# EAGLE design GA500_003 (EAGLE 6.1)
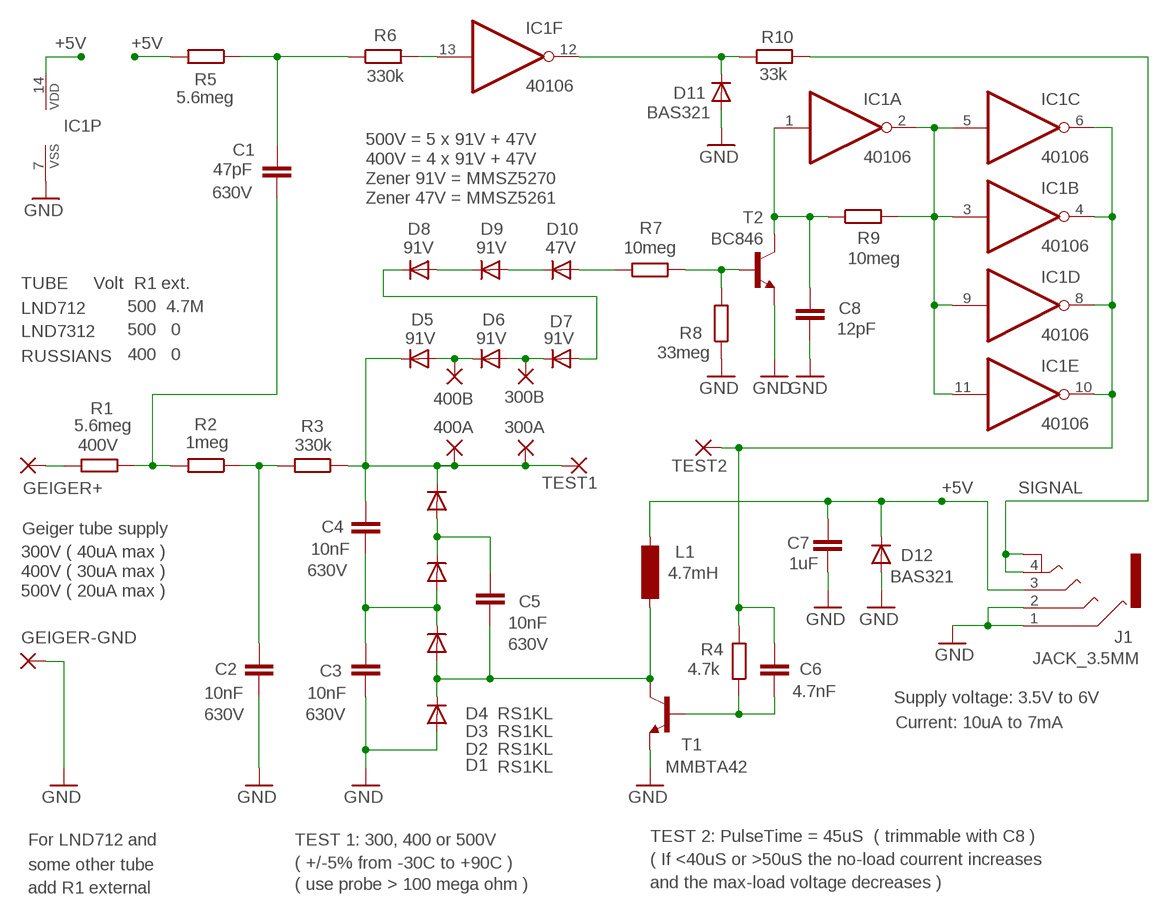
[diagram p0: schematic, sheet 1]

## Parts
300A  TEST  WIREPADSMD1,00-1,00  [SMD1,00-1,00]
300B  TEST  WIREPADSMD1,00-1,00  [SMD1,00-1,00]
400A  TEST  WIREPADSMD1,00-1,00  [SMD1,00-1,00]
400B  TEST  WIREPADSMD1,00-1,00  [SMD1,00-1,00]
C1  47pF  C-EUC1206  [C1206]
C2  10nF  C-EUC1206  [C1206]
C3  10nF  C-EUC1206  [C1206]
C4  10nF  C-EUC1206  [C1206]
C5  10nF  C-EUC1206  [C1206]
C6  4.7nF  C-EUC0603  [C0603]
C7  1uF  C-EUC0603  [C0603]
C8  12pF  C-EUC0603  [C0603]
D1  RS1KL  DIODE-SOD123-LARGE  [SOD123-LARGE]
D2  RS1KL  DIODE-SOD123-LARGE  [SOD123-LARGE]
D3  RS1KL  DIODE-SOD123-LARGE  [SOD123-LARGE]
D4  RS1KL  DIODE-SOD123-LARGE  [SOD123-LARGE]
D5  MMSZ5270  DIODE-SOD123  [SOD123]
D6  MMSZ5270  DIODE-SOD123  [SOD123]
D7  MMSZ5270  DIODE-SOD123  [SOD123]
D8  MMSZ5270  DIODE-SOD123  [SOD123]
D9  MMSZ5270  DIODE-SOD123  [SOD123]
D10  MMSZ5261  DIODE-SOD123-LARGE  [SOD123-LARGE]
D11  BAS321  DIODE-SOD323  [SOD323]
D12  BAS321  DIODE-SOD323  [SOD323]
GEIGER+  Geiger tube supply  WIREPADSMD2,54-3,81  [SMD2,54-3,81]
GEIGER-GND  1.6mm  WIREPADSMD2,54-3,81  [SMD2,54-3,81]
IC1  40106  40106SOIC  [SOIC14_S]
J1  JACK_3.5MM  JACK_3.5MM_SMD_4JACK4  [JACK_4]
L1  4.7mH  INDUCTOR_4.7MH472KU  [MSD75]
R1  5.6meg  R-EU_R1206  [R1206]
R2  1meg  R-EU_R1206  [R1206]
R3  330k  R-EU_R1206  [R1206]
R4  4.7k  R-EU_R0603  [R0603]
R5  5.6meg  R-EU_R1206  [R1206]
R6  330k  R-EU_R1206  [R1206]
R7  10meg  R-EU_R1206_L  [R1206_L]
R8  33meg  R-EU_R0603  [R0603]
R9  10meg  R-EU_R0603  [R0603]
R10  33k  R-EU_R0603  [R0603]
T1  MMBTA42  -NPN-BC846  [SOT23_L]
T2  BC846  BC846L  [SOT23_L]
TEST1  TEST  WIREPADSMD1,27-2,54  [SMD1,27-2,54]
TEST2  TEST  WIREPADSMD1,27-2,54  [SMD1,27-2,54]

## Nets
+5V: C7.1 D12.C IC1.14(P:VDD) J1.3 L1.1 R5.2
DATA: C1.1 R5.1 R6.1
GND: C2.1 C3.1 C7.2 C8.2 D1.A D11.A D12.A GEIGER-GND.1(P) IC1.7(P:VSS) J1.1 J1.2 R8.1 T1.2(E) T2.2(E)
N$1: C6.1 R4.1 T1.1(B)
N$2: C6.2 IC1.4(B:O) IC1.6(C:O) IC1.8(D:O) IC1.10(E:O) R4.2 TEST2.1(P)
N$3: C3.2 C4.1 D2.C D3.A
N$4: C2.2 R2.1 R3.2
N$5: GEIGER+.1(P) R1.1
N$6: IC1.2(A:O) IC1.3(B:I) IC1.5(C:I) IC1.9(D:I) IC1.11(E:I) R9.2
N$7: D10.A R7.1
N$8: D7.A D8.C
N$9: IC1.13(F:I) R6.2
N$10: 300A.1(P) 400A.1(P) C4.2 D4.C D5.C R3.1 TEST1.1(P)
N$11: C8.1 IC1.1(A:I) R9.1 T2.3(C)
N$12: D8.A D9.C
N$13: 400B.1(P) D5.A D6.C
N$14: C1.2 R1.2 R2.2
N$15: D11.C IC1.12(F:O) R10.1
N$16: 300B.1(P) D6.A D7.C
N$17: C5.2 D3.C D4.A
N$18: D9.A D10.C
N$20: R7.2 R8.2 T2.1(B)
N$21: C5.1 D1.C D2.A L1.2 T1.3(C)
SIGNAL: J1.4 J1.4@1 R10.2

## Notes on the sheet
- 500V = 5 x 91V + 47V
- 400V = 4 x 91V + 47V
- Zener 91V = MMSZ5270
- Zener 47V = MMSZ5261
- TUBE     Volt  R1 ext.
- LND712 | 500  4.7M
- LND7312 | 500   0
- RUSSIANS | 400   0
- 300V ( 40uA max )
- 400V ( 30uA max )
- 500V ( 20uA max )
- Supply voltage: 3.5V to 6V
- Current: 10uA to 7mA
- For LND712 and | TEST 1: 300, 400 or 500V | TEST 2: PulseTime = 45uS  ( trimmable with C8 )
- ( +/-5% from -30C to +90C ) | ( If <40uS or >50uS the no-load courrent increases
- some other tube
- ( use probe > 100 mega ohm ) | and the max-load voltage decreases )
- add R1 external

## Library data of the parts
300A 300B 400A 400B GEIGER+ GEIGER-GND TEST1 TEST2 = 00-LIVIO:WIREPAD: Wire PAD connect wire on PCB
C1-C5 = 00-LIVIO:C-EU: CAPACITOR, European symbol; VOLTAGE: 630V
C6-C8 = 00-LIVIO:C-EU: CAPACITOR, European symbol
D1-D4 D11 D12 = 00-LIVIO:DIODE-: DIODE
D5-D9 = 00-LIVIO:DIODE-: DIODE; VZ: 91V
D10 = 00-LIVIO:DIODE-: DIODE; VZ: 47V
IC1 = 00-LIVIO:40106: Hex SCHMITT TRIGGER 40106 74C14
J1 = 00-LIVIO:JACK_3.5MM_SMD_4: Jack 4 poles SMD 3.5mm - Lumberg RC-5325A - Farnell 1368640
L1 = 00-LIVIO:INDUCTOR_4.7MH: INDUCTOR
R1 = 00-LIVIO:R-EU_: RESISTOR, European symbol; VOLTAGE: 400V
R2-R10 = 00-LIVIO:R-EU_: RESISTOR, European symbol
T1 = 00-LIVIO:*-NPN-: NPN Transistror
T2 = 00-LIVIO:BC846

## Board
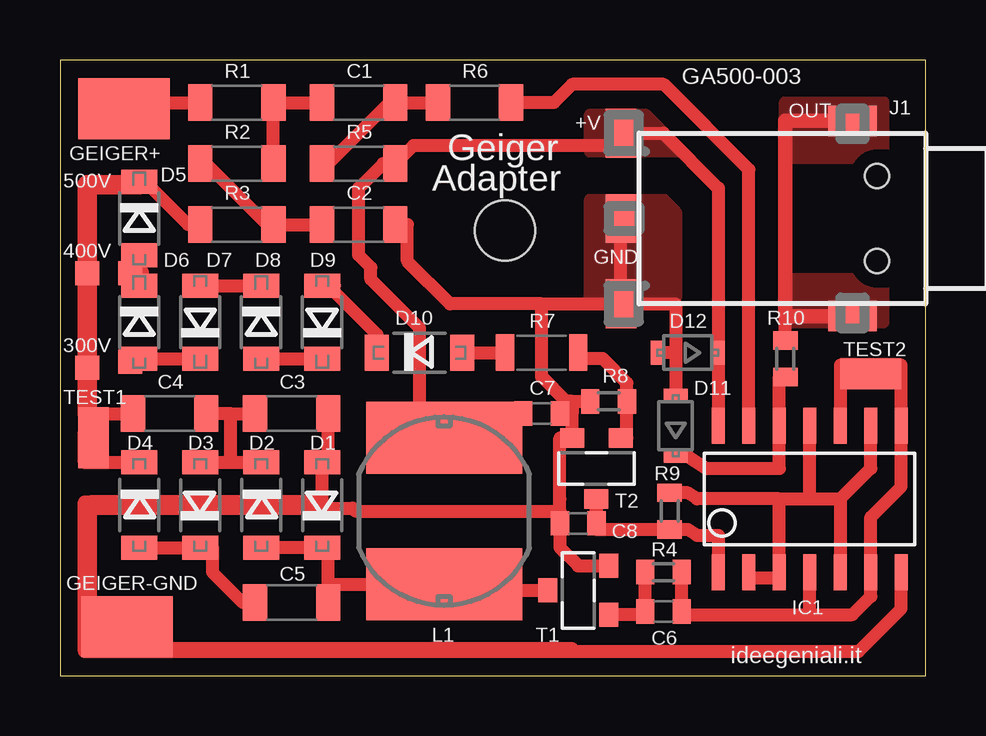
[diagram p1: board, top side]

Size 36.07 x 25.65 mm. Coordinates in mm from the lower left corner, seen from the top.
Outline: 0,0 36.07,0 36.07,25.65 0,25.65 0,0
Copper layers (1*16): Top 0.035mm / dielectric 1.5mm / Bottom 0.035mm
Design rules: minimum track width 10mil, minimum drill 23mil, track to track 23mil, track to pad 23mil, pad to pad 23mil, via to via 23mil, smd to smd 23mil, copper to edge 23mil, drill to drill 8mil, minimum pad ring 5mil, minimum via ring 8mil, stop-mask expansion 4mil, vias tented up to drill 0mil, thermal gap 35mil
Holes 2.5 mm at 18.54,18.54

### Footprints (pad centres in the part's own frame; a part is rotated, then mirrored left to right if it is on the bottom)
SMD1,00-1,00 = smd 1 x 1: 1 0,0
C1206 = smd 1.016 x 1.524: 1 -1.524,0; 2 1.524,0
C0603 = smd 0.762 x 1.016: 1 -0.762,0; 2 0.762,0
SOD123-LARGE = smd 1 x 1.5: A 1.778,0; C -1.778,0
SOD123 = smd 1 x 1.5: A 1.524,0; C -1.524,0
SOD323 = smd 0.55 x 1: A 1.27,0; C -1.27,0
SMD2,54-3,81 = smd 2.54 x 3.81: 1 0,0
SOIC14_S = smd 0.55 x 1.5: 1 -3.81,-3.048; 2 -2.54,-3.048; 3 -1.27,-3.048; 4 0,-3.048; 5 1.27,-3.048; 6 2.54,-3.048; 7 3.81,-3.048; 8 3.81,3.048; 9 2.54,3.048; 10 1.27,3.048; 11 0,3.048; 12 -1.27,3.048; 13 -2.54,3.048; 14 -3.81,3.048
JACK_4 = smd 2.032 x 1.27: 1 0,6.604; 2 -3.556,6.604; 3 3.556,6.604 | smd 1.27 x 2.032: 4 4.064,-3.048; 4@1 -4.064,-3.048 | hole 1: 1.778,-4.064; -1.778,-4.064
MSD75 = smd 3 x 6.5: 1 3.048,0; 2 -3.048,0
R1206 = smd 1.016 x 1.524: 1 -1.524,0; 2 1.524,0
R0603 = smd 0.762 x 1.016: 1 -0.762,0; 2 0.762,0
R1206_L = smd 0.762 x 1.524: 1 -1.524,0; 2 1.524,0
SOT23_L = smd 1 x 0.8: 1 -1.016,-1.27; 2 1.016,-1.27; 3 0,1.27
SMD1,27-2,54 = smd 1.27 x 2.54: 1 0,0

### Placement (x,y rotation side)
300A  1.14,16.76 0 top
300B  2.92,13.08 90 top
400A  1.14,12.83 0 top
400B  2.92,16.76 0 top
C1  12.45,23.88 180 top
C2  12.45,18.8 180 top
C3  9.65,10.92 180 top
C4  4.57,10.92 180 top
C5  9.65,3.05 180 top
C6  25.15,2.67 0 top
C7  20.07,10.92 0 top
C8  21.59,6.35 180 top
D1  10.92,7.11 90 top
D2  8.38,7.11 270 top
D3  5.84,7.11 90 top
D4  3.3,7.11 270 top
D5  3.3,19.05 270 top
D6  3.3,14.73 270 top
D7  5.84,14.73 90 top
D8  8.38,14.73 270 top
D9  10.92,14.73 90 top
D10  14.99,13.46 0 top
D11  25.65,10.41 90 top
D12  26.16,13.46 180 top
GEIGER+  2.67,23.62 90 top
GEIGER-GND  2.79,2.03 270 top
IC1  31.24,7.37 0 top
J1  29.97,19.05 90 top
L1  16,6.86 90 top
R1  7.37,23.88 0 top
R2  7.37,21.34 0 top
R3  7.37,18.8 0 top
R4  25.15,4.32 0 top
R5  12.45,21.34 0 top
R6  17.27,23.88 0 top
R7  20.07,13.46 0 top
R8  22.86,11.43 0 top
R9  25.4,6.86 90 top
R10  30.23,13.21 90 top
T1  21.59,3.56 90 top
T2  22.35,8.64 180 top
TEST1  1.4,9.91 0 top
TEST2  33.78,12.57 90 top

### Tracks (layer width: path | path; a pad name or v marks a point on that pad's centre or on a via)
+5V
  Top 0.55: C7.1 16,10.92 L1.1 14.99,9.91 14.99,14.48 12.95,16.51 12.95,17.02 12.45,17.53 12.45,20.32 13.46,21.34 R5.2 14.73,22.1 23.37,22.1 J1.3 25.15,22.61 27.43,20.32 D12.C IC1.14
  pour Top (isolate 0.1, rank 6, no thermals): 22.1,23.37 24.38,23.37 25.91,21.84 22.1,21.84
DATA
  Top 0.55: R5.1 11.18,21.34 13.72,23.88 C1.1 R6.1
GND
  Top 0.55: IC1.7 35.05,2.79 33.27,1.02 2.79,1.02 | 2.79,1.02 2.79,1.14 | 2.79,1.14 GEIGER-GND.1 2.79,1.14 | 2.79,1.02 1.02,1.02 1.02,6.99 | 2.79,1.02 2.79,1.14 | 1.02,6.99 1.02,7.24 1.27,7.24 | 10.92,7.24 1.27,7.24 | T1.2 21.59,4.57 20.83,5.33 C8.2 | 20.83,6.86 20.83,7.37 20.83,9.91 T2.2 21.34,11.43 | J1.2 J1.1 | C3.1 11.18,8.89 D1.A 10.92,7.24 | 10.92,6.99 10.92,7.24 | 10.92,6.99 12.19,6.99 12.32,6.86 20.83,6.86 | 20.83,6.86 20.83,6.6 | 20.83,6.6 C8.2 | 21.34,11.43 R8.1 | 21.34,11.43 21.34,10.92 C7.2 | 21.34,11.43 21.08,11.43 20.07,12.45 20.07,15.49 | 25.65,13.46 25.65,15.49 J1.2 | 25.65,13.46 D11.A | C2.1 14.48,18.8 14.48,17.27 16.26,15.49 20.07,15.49 | 20.07,15.49 J1.2 | 25.65,13.46 D12.A | 1.27,7.24 1.27,3.3 | 1.02,6.99 10.92,6.99 | 20.83,6.6 C8.2 | 2.79,1.14 21.34,1.14 | 2.79,1.14 2.79,1.02
  pour Top (isolate 0.1, rank 6, no thermals): 22.1,19.81 25.15,19.81 25.65,19.3 25.65,15.75 22.1,15.75
N$1
  Top 0.55: T1.1 24.38,2.54 C6.1 R4.1
N$2
  Top 0.55: 32.51,12.95 32.51,12.7 IC1.10 | 33.78,12.95 34.54,12.95 35.05,12.95 IC1.8 35.05,7.87 33.78,6.6 IC1.6 33.78,3.3 33.02,2.54 31.24,2.54 | 33.78,12.95 32.51,12.95 | 31.24,2.54 IC1.4 | R4.2 C6.2 25.91,2.54 31.24,2.54 | 33.78,12.95 32.51,12.95 | 33.78,12.95 TEST2.1
N$3
  Top 0.55: 7.11,10.92 C3.2 | 7.11,8.89 7.11,10.92 | 7.11,10.92 C4.1 | D3.A 7.11,8.89 | 7.11,8.89 D2.C
N$4
  Top 0.55: R2.1 6.1,21.34 8.64,18.8 R3.2 C2.2
N$5
  Top 0.55: GEIGER+.1 2.67,23.88 R1.1
N$6
  Top 0.55: 31.24,7.37 IC1.11 | 32.51,7.37 33.78,8.64 IC1.9 | 32.51,7.37 IC1.5 | 29.97,7.37 31.24,7.37 | 31.24,7.37 32.51,7.37 | IC1.2 28.7,4.06 29.97,4.06 IC1.3 29.97,7.37 | R9.2 26.16,7.62 26.54,7.37 29.97,7.37
N$7
  Top 0.55: D10.A R7.1
N$8
  Top 0.55: D7.A D8.C
N$9
  Top 0.55: IC1.13 28.7,21.08 25.15,24.64 21.34,24.64 20.57,23.88 R6.2
N$10
  Top 0.55: D4.C 1.02,8.89 1.02,10.16 | 1.02,10.16 1.14,10.16 | 1.14,10.16 1.14,10.92 C4.2 | D5.C 3.56,20.57 5.33,18.8 R3.1 | 1.02,10.16 1.14,10.16 | 1.14,10.16 TEST1.1
  Top 0.813: 400A.1 1.14,10.92 400A.1 | 400A.1 300A.1 | 300A.1 1.14,20.45 3.3,20.45 D5.C | 300A.1 400A.1
N$11
  Top 0.55: IC1.1 27.43,5.33 27.43,5.84 26.54,5.84 26.16,6.1 R9.1 24.13,6.1 22.35,6.1 T2.3 C8.1
N$12
  Top 0.55: D8.A D9.C
N$13
  Top 0.55: 3.3,16.76 3.3,17.27
  Top 0.61: D6.C 3.3,16.51 3.3,16.76 3.3,17.27 D5.A
  Top 0.813: 400B.1 3.3,16.76
N$14
  Top 0.55: R2.2 R1.2 C1.2
N$15
  Top 0.55: D11.C 26.16,9.14 26.92,8.64 29.97,8.64 IC1.12 29.97,12.45 R10.1
N$16
  Top 0.55: D6.A D7.C
  Top 0.813: 300B.1 3.3,13.08 D6.A
N$17
  Top 0.55: D4.A D3.C 6.35,5.33 6.35,4.32 7.62,3.05 C5.2
N$18
  Top 0.55: D9.A 11.43,16.26 11.43,16 13.21,14.22 D10.C
N$20
  Top 0.55: T2.1 23.62,9.91 R8.2 23.62,12.19 22.61,13.21 21.59,13.21 R7.2
N$21
  Top 0.55: C5.1 11.18,3.81 | D2.A D1.C 11.18,5.33 11.18,3.81 | T1.3 16,3.56 L1.2 11.18,3.81
SIGNAL
  Top 0.55: R10.2 30.23,14.99
  Top 0.6: J1.4 30.23,23.11 30.23,14.99 J1.4@1
  pour Top (isolate 0.1, rank 6, no thermals): 30.23,23.88 34.29,23.88 34.29,21.59 30.23,21.59
  pour Top (isolate 0.1, rank 6, no thermals): 30.23,16.51 34.29,16.51 34.29,14.73 30.23,14.73

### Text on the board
tNames: GA500-003 | +V | OUT | Geiger | 500V | Adapter | 400V | GND | 300V | ideegeniali.it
